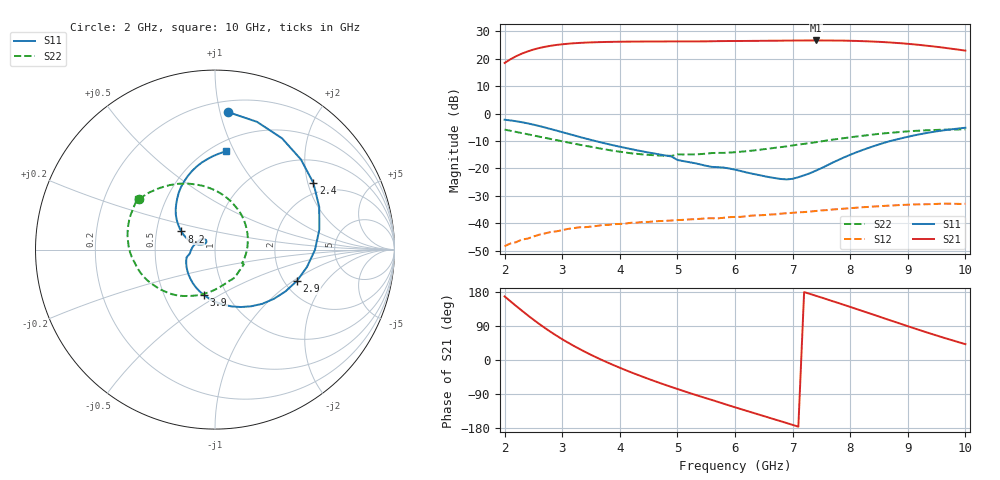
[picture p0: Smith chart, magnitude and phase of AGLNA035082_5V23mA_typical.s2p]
! Keysight Technologies,N5245B,MY58421923,A.15.40.11
! pna-50_lab Wed Jul 27 17:21:22 2022
# HZ S DB R 50
!freq (Hz)  S11DB  S11A  S21DB  S21A  S12DB  S12A  S22DB  S22A
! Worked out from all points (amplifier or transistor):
!   81 points, 2 GHz to 10 GHz, reference 50 ohm
!   highest |S21| = 26.7 dB at 7.4 GHz (marker M1)
!   |S21| within 3 dB of that: 2.558 GHz to 9.752 GHz (7.195 GHz wide, 117 % of centre)
!   unconditionally stable (mu >= 1): start of sweep to 9.427 GHz
!   at 3.3 GHz: K = 2.50, MAG = 26.8 dB, |S12| = -41.5 dB
!   at 6 GHz: K = 1.90, MAG = 26.7 dB, |S12| = -37.7 dB
!   at 10 GHz: K = 1.00, MSG = 28.0 dB, |S12| = -32.9 dB
!   lowest NFmin = 0.67 dB at 5.9 GHz
!   S11 on the Smith chart (normalised r, x): 2 GHz: 0.28, +1.06; 2.4 GHz: 1.64, +2.17; 2.9 GHz: 2.34, -1.07; 3.9 GHz: 0.78, -0.43; 8.2 GHz: 0.67, +0.14; 10 GHz: 0.59, +0.92
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2e9  -2.27 84.8  18.47 167.8  -48.41 94.0  -5.87 146.3
2.2e9  -2.81 58.9  20.92 142.5  -46.95 90.1  -6.71 131.9
2.4e9  -3.58 34.2  22.67 118.1  -45.65 84.4  -7.56 118.7
2.6e9  -4.55 10.9  23.91 95.2  -44.23 79.5  -8.43 106.5
2.9e9  -6.21 -20.8  25.03 64.3  -43.01 67.9  -9.70 88.7
3.2e9  -7.94 -48.8  25.64 37.3  -41.82 59.0  -10.95 71.7
3.4e9  -9.09 -65.7  25.89 21.3  -41.48 53.4  -11.77 60.4
3.6e9  -10.16 -81.3  26.03 6.4  -41.02 47.8  -12.54 49.0
3.9e9  -11.66 -103.3  26.18 -14.0  -40.37 40.6  -13.61 31.8
4.3e9  -13.43 -129.9  26.27 -38.6  -39.81 32.8  -14.72 8.0
4.7e9  -14.98 -154.1  26.29 -60.9  -39.24 25.6  -15.33 -15.2
5.3e9  -18.11 171.8  26.33 -91.4  -38.55 14.6  -14.91 -41.4
6e9  -20.49 142.2  26.47 -124.8  -37.73 5.8  -14.12 -72.0
6.7e9  -23.58 136.1  26.58 -157.3  -36.79 -4.5  -12.49 -96.8
7.1e9  -23.23 153.5  26.66 -176.0  -36.07 -11.2  -11.33 -110.3
7.4e9  -20.88 161.7  26.67 169.7  -35.58 -15.9  -10.48 -120.3
7.8e9  -16.90 161.7  26.62 150.2  -34.89 -23.3  -9.23 -134.0
8.2e9  -13.43 151.6  26.43 129.9  -34.22 -31.4  -8.16 -148.6
8.7e9  -10.02 133.9  25.92 104.4  -33.59 -43.1  -7.03 -166.9
9e9  -8.49 122.4  25.45 89.3  -33.29 -50.4  -6.51 -177.8
9.4e9  -6.84 106.5  24.59 69.5  -33.08 -59.9  -6.05 167.4
1e10  -5.19 83.9  22.96 41.8  -32.94 -74.6  -5.77 147.0
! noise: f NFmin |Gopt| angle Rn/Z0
2e+09  1.547  0.3904  -146.9  0.1701
2.9e+09  1.267  0.02563  -36.41  0.2926
3.7e+09  0.9864  0  90  0.06375
4.6e+09  0.8013  0.143  -15.73  0.2512
5.6e+09  0.7315  0.1157  -63.34  0.3828
6.6e+09  0.7963  0.1135  -178.7  0.1463
7.5e+09  0.8238  0  90  0.05221
8.3e+09  0.8694  0.08609  -4.776  0.3662
9.1e+09  0.9174  0  90  0.0588
1e+10  1.069  0.09752  -128.4  0.2452
